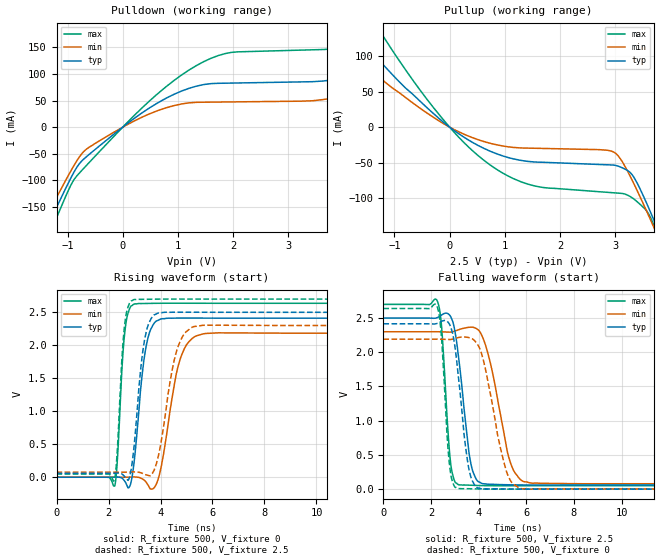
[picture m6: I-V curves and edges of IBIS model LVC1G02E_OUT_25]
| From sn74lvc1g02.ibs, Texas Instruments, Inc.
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[Model]   LVC1G02E_OUT_25
Model_type  Output
Vref =   0
Rref =   500
Cref =   30p
Vmeas =   1.25
| variable   typ   min   max
C_comp   7.23pF   3.05pF   13.59pF
| C_pullup   5.96pF   3.16pF   8.27pF
| C_pulldown   8.50pF   3.05pF   13.59pF
[Temperature Range]   40   100   -40
| Ambient temperature   25   85   -40
[Voltage range]   2.5   2.3   2.7
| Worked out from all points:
|   slope of the pulldown table from 0 to 0.375 V, typ, clamps not added: 13.1 ohm
|   slope of the pullup table from 0 to 0.375 V, typ, clamps not added: 19.1 ohm
|   rising waveform, R_fixture 500, V_fixture 0: 20-80 % time 371ps typ, 572ps min, 224ps max; typ from 0 V to 2.41 V
|   falling waveform, R_fixture 500, V_fixture 2.5: 20-80 % time 462ps typ, 738ps min, 282ps max; typ from 2.5 V to 0.06 V
|   rising waveform, R_fixture 500, V_fixture 2.5: 20-80 % time 356ps typ, 561ps min, 222ps max; typ from 0.06 V to 2.5 V
|   falling waveform, R_fixture 500, V_fixture 0: 20-80 % time 445ps typ, 742ps min, 268ps max; typ from 2.42 V to 0 V
[Pulldown]
| LVC1G02E_OUT_25
|   Voltage   I(typ)   I(min)   I(max)
-5.5V     -1.088A    -986.7mA   -1.218A
-1.56V    -231.1mA   -204.2mA   -260.3mA
-1.17V    -144.5mA   -126.4mA   -163.1mA
-660mV    -55.82mA   -41.58mA   -72.25mA
490mV     36.46mA    25.18mA    49.68mA
1.47V     80.07mA    46.85mA    123.2mA
3.845V    90.17mA    55.74mA    148mA
5.345V    157.8mA    105.8mA    231.8mA
5.905V    188.7mA    52.63mA    282.3mA
6.525V    93.57mA    53.14mA    298.9mA
7.56V     94.12mA    54.12mA    160.7mA
11V       99.65mA    57.57mA    168.9mA
[Pullup]
| LVC1G02E_OUT_25
|   Voltage   I(typ)   I(min)   I(max)
-5.5V     550.8mA    435.9mA    767.8mA
-2.33V    193.1mA    147.8mA    276mA
-1.875V   148.5mA    112.7mA    213.7mA
-1.315V   97.46mA    72.94mA    141.6mA
-185mV    11.74mA    8.463mA    17.18mA
705mV     -32.88mA   -22.14mA   -51.6mA
1.55V     -49.14mA   -29.77mA   -83mA
2.98V     -53.5mA    -35.34mA   -92.52mA
3.31V     -67.24mA   -74.95mA   -99.61mA
3.58V     -108.8mA   -119.9mA   -118.8mA
3.73V     -136mA     -146.2mA   -142.9mA
11V       -1.654A    -1.558A    -1.795A
[Ramp]
| LVC1G02E_OUT_25
| variable   typ   min   max
dV/dt_r   1.54/4.06E-10   1.42/6.35E-10   1.66/2.38E-10
dV/dt_f   1.51/4.92E-10   1.37/7.72E-10   1.64/2.98E-10
R_load = 500
[Rising Waveform]
| LVC1G02E_OUT_25
R_fixture =   500
C_fixture =   0
L_fixture =   0
V_fixture =   0
V_fixture_min = 0
V_fixture_max = 0
|   Time   V(typ)   V(min)   V(max)
0s        123.6pV    5.747nV    2.756nV
2.24ns    583.5uV    -29.22uV   -132.3mV
2.62ns    -58.19mV   -103.5uV   2.177V
2.82ns    -134.3mV   1.674mV    2.564V
3ns       283.7mV    4.456mV    2.627V
3.45ns    1.991V     -76.6mV    2.634V
4.035ns   2.401V     176.7mV    2.637V
4.745ns   2.413V     1.777V     2.638V
5.615ns   2.412V     2.171V     2.637V
24.99ns   2.411V     2.183V     2.637V
[Falling Waveform]
| LVC1G02E_OUT_25
R_fixture =   500
C_fixture =   0
L_fixture =   0
V_fixture =   2.5
V_fixture_min = 2.3
V_fixture_max = 2.7
|   Time   V(typ)   V(min)   V(max)
0s        2.5V       2.3V       2.7V
2.27ns    2.508V     2.3V       2.744V
2.445ns   2.545V     2.299V     2.366V
2.815ns   2.525V     2.295V     403.7mV
3.16ns    1.916V     2.33V      62.59mV
3.595ns   527.1mV    2.365V     57.61mV
3.88ns    155.2mV    2.35V      53.83mV
5.3ns     62.86mV    422.2mV    48.86mV
5.895ns   60.43mV    109.1mV    49.11mV
24.99ns   60.11mV    77.11mV    49.35mV
[Rising Waveform]
| LVC1G02E_OUT_25
R_fixture =   500
C_fixture =   0
L_fixture =   0
V_fixture =   2.5
V_fixture_min = 2.3
V_fixture_max = 2.7
|   Time   V(typ)   V(min)   V(max)
0s        60.06mV    77.04mV    49.31mV
2.225ns   60.39mV    77.02mV    -40.85mV
2.61ns    14.39mV    76.94mV    2.274V
2.98ns    458mV      81.61mV    2.693V
3.29ns    1.821V     61.23mV    2.697V
3.555ns   2.337V     24.83mV    2.698V
3.925ns   2.491V     335.3mV    2.7V
4.625ns   2.501V     1.922V     2.701V
5.295ns   2.501V     2.285V     2.7V
24.99ns   2.5V       2.3V       2.7V
[Falling Waveform]
| LVC1G02E_OUT_25
R_fixture =   500
C_fixture =   0
L_fixture =   0
V_fixture =   0
V_fixture_min = 0
V_fixture_max = 0
|   Time   V(typ)   V(min)   V(max)
0s        2.416V     2.191V     2.64V
2.25ns    2.421V     2.192V     2.673V
2.43ns    2.451V     2.191V     2.257V
2.775ns   2.409V     2.187V     357.3mV
3.13ns    1.699V     2.213V     7.671mV
3.505ns   477.1mV    2.22V      5.899mV
3.805ns   74mV       2.177V     3.654mV
5.175ns   1.822mV    248.9mV    -310.4uV
5.765ns   128.1uV    8.002mV    -150.5uV
24.99ns   41.59uV    58.04uV    34.85uV
